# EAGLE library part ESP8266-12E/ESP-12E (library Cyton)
ESP-12E WiFi Module
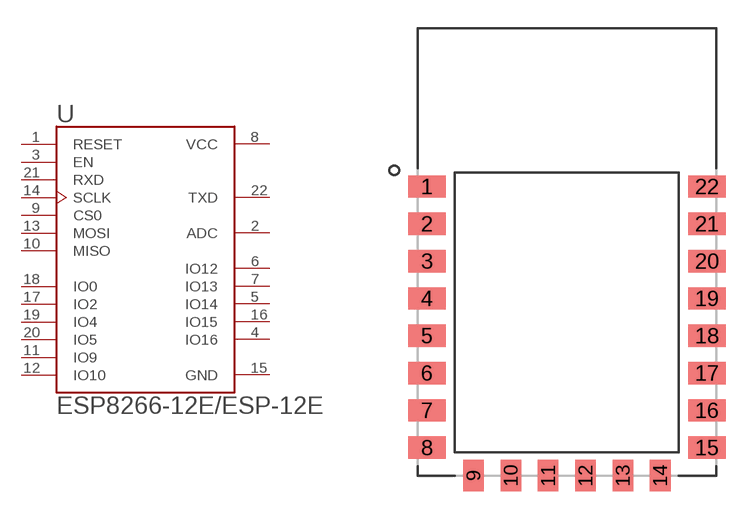
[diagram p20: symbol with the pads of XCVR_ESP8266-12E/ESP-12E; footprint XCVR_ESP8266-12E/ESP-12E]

Designator prefix U

## ESP8266-12E/ESP-12E (AVAILABILITY: Unavailable; DESCRIPTION: This WiFi module has a 32-bit MCU micro and clock speeds supporting 80 MHz or 160 MHz. Supports the RTOS and integrated Wi-Fi MAC/BB/RF/PA/LNA, and has an on-board antenna.; MF: AI-Thinker; MP: ESP8266-12E/ESP-12E; PACKAGE: None; PRICE: None)  [XCVR_ESP8266-12E/ESP-12E]
1  RESET  in
2  ADC  pas
3  EN  in
4  IO16
5  IO14
6  IO12
7  IO13
8  VCC  pwr
9  CS0  in
10  MISO
11  IO9
12  IO10
13  MOSI
14  SCLK  in
15  GND  pwr
16  IO15
17  IO2
18  IO0
19  IO4
20  IO5
21  RXD  in
22  TXD  out

## Footprint XCVR_ESP8266-12E/ESP-12E (pad centres in mm)
smd 2 x 1.2: 1 -7.5,7; 2 -7.5,5; 3 -7.5,3; 4 -7.5,1; 5 -7.5,-1; 6 -7.5,-3; 7 -7.5,-5; 8 -7.5,-7; 15 7.5,-7; 16 7.5,-5; 17 7.5,-3; 18 7.5,-1; 19 7.5,1; 20 7.5,3; 21 7.5,5; 22 7.5,7
smd 1.1 x 1.7: 9 -5,-8.5; 10 -3,-8.5; 11 -1,-8.5; 12 1,-8.5; 13 3,-8.5; 14 5,-8.5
